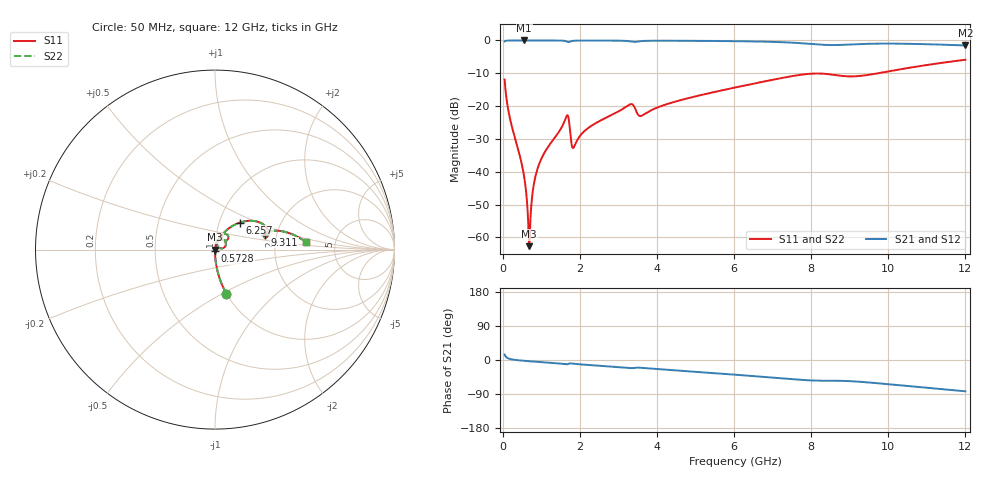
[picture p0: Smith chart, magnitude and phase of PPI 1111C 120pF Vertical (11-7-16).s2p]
# GHz S MA R 50
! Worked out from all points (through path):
!   1601 points, 50 MHz to 12 GHz, reference 50 ohm
!   highest |S21| = -0.01 dB at 557.9 MHz (marker M1); lowest = -1.5 dB at 12 GHz (marker M2)
!   group delay of S21, straight-line fit = 18.9 ps
!   lowest |S11| = -62.7 dB at 684.8 MHz (marker M3), VSWR 1.00, Z = 50.1 - j0.025 ohm
!   |S11| at or under -10 dB: start of sweep to 9.736 GHz
!   |S22| runs from -62.7 to -5.9 dB; largest |S21 - S12| = 0
!   S11 on the Smith chart (normalised r, x): 50 MHz: 1.00, -0.53; 572.8 MHz: 1.00, -0.01; 6.257 GHz: 1.25, +0.39; 9.311 GHz: 1.73, +0.31; 12 GHz: 3.02, +0.34
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0.05  0.2544 -75.4  0.9669 14.5  0.9669 14.5  0.2544 -75.4
0.1844375  0.06647 -86.7  0.9974 2.9  0.9974 2.9  0.06647 -86.7
0.557875  0.008287 -87.7  0.9993 -2.2  0.9993 -2.2  0.008287 -87.7
0.5728125  0.007248 -87.2  0.9993 -2.3  0.9993 -2.3  0.007248 -87.2
0.6475  0.002505 -77.1  0.9993 -2.9  0.9993 -2.9  0.002505 -77.1
0.6848437  0.0007338 -19.9  0.9993 -3.2  0.9993 -3.2  0.0007338 -19.9
0.7221875  0.002018 65.5  0.9992 -3.5  0.9992 -3.5  0.002018 65.5
0.7894062  0.005498 78.0  0.9992 -4.0  0.9992 -4.0  0.005498 78.0
0.856625  0.008843 80.3  0.9991 -4.5  0.9991 -4.5  0.008843 80.3
1.118031  0.02108 80.7  0.9987 -6.5  0.9987 -6.5  0.02108 80.7
1.655781  0.07002 52.5  0.9671 -11.4  0.9671 -11.4  0.07002 52.5
1.827562  0.02298 42.9  0.9857 -9.6  0.9857 -9.6  0.02298 42.9
2.044156  0.03748 72.2  0.9952 -11.7  0.9952 -11.7  0.03748 72.2
3.291437  0.1054 56.0  0.9714 -21.3  0.9714 -21.3  0.1054 56.0
3.57525  0.07047 50.5  0.9746 -20.5  0.9746 -20.5  0.07047 50.5
4.038312  0.09652 62.5  0.9898 -24.3  0.9898 -24.3  0.09652 62.5
6.025  0.1916 49.3  0.9747 -38.7  0.9747 -38.7  0.1916 49.3
6.256531  0.2046 47.3  0.9708 -40.5  0.9708 -40.5  0.2046 47.3
8.019156  0.312 23.1  0.8826 -54.0  0.8826 -54.0  0.312 23.1
9.31125  0.2897 16.7  0.8825 -57.8  0.8825 -57.8  0.2897 16.7
10.01331  0.3382 17.9  0.8942 -64.0  0.8942 -64.0  0.3382 17.9
12  0.508 4.7  0.8375 -82.6  0.8375 -82.6  0.508 4.7
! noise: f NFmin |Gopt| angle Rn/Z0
0.05  0.0003509  0.8586  0.4116  0.0005309
1.372  0.004954  0.7428  6.374  0.003854
2.701  0.00842  0.7099  12.44  0.005648
4.031  0.01421  0.7418  18.52  0.01076
5.36  0.01495  0.6889  24.11  0.008952
6.682  0.02679  0.7767  30.12  0.02291
8.012  0.07324  0.8978  36.12  0.1416
9.341  0.08172  0.896  41.61  0.15
10.67  0.05812  0.8425  46.64  0.06609
12  0.05176  0.8109  51.35  0.04648
